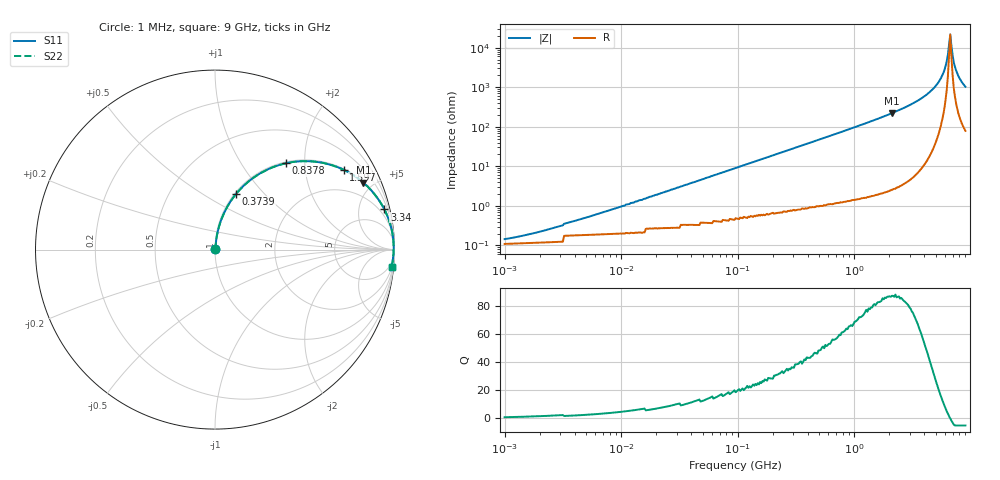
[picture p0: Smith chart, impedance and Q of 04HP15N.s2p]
# MHz S MA R 50
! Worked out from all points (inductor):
!   396 points, 1 MHz to 9 GHz, reference 50 ohm
!   read as one part in series: L = 15 nH near 6.037 MHz
!   highest Q = 87 at 2.107 GHz (marker M1), where L = 16.7 nH
!   self-resonance near 6.518 GHz
!   S11 on the Smith chart (normalised r, x): 1 MHz: 1.00, +0.00; 373.9 MHz: 1.02, +0.71; 837.8 MHz: 1.03, +1.60; 1.597 GHz: 1.04, +3.19; 3.34 GHz: 1.11, +8.41; 9 GHz: 3, -21
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1  0.001508 38.6  0.999 -0.1  0.999 -0.1  0.001508 38.6
1.997  0.00231 54.3  0.999 -0.1  0.999 -0.1  0.00231 54.3
4.578  0.004607 69.0  0.998 -0.2  0.998 -0.2  0.004607 69.0
20.961  0.02 81.3  0.997 -1.1  0.997 -1.1  0.02 81.3
95.968  0.09 81.9  0.991 -5.1  0.991 -5.1  0.09 81.9
373.904  0.331 69.3  0.936 -19.3  0.936 -19.3  0.331 69.3
439.375  0.381 66.3  0.916 -22.4  0.916 -22.4  0.381 66.3
837.792  0.621 50.7  0.774 -38.4  0.774 -38.4  0.621 50.7
1597.486  0.843 31.9  0.528 -57.5  0.528 -57.5  0.843 31.9
2011.613  0.898 25.5  0.43 -63.9  0.43 -63.9  0.898 25.5
2106.521  0.907 24.3  0.411 -65.1  0.411 -65.1  0.907 24.3
3340.263  0.97 13.3  0.231 -75.9  0.231 -75.9  0.97 13.3
4612.443  0.99 6.8  0.119 -81.6  0.119 -81.6  0.99 6.8
5546.474  0.995 3.4  0.059 -83.0  0.059 -83.0  0.995 3.4
5943.595  0.995 2.1  0.037 -81.7  0.037 -81.7  0.995 2.1
6224.015  0.996 1.3  0.022 -77.8  0.022 -77.8  0.996 1.3
6369.149  0.996 0.8  0.015 -72.6  0.015 -72.6  0.996 0.8
6669.648  0.995 -0.0  0.004608 0.9  0.004608 0.9  0.995 -0.0
6984.324  0.995 -0.8  0.015 70.6  0.015 70.6  0.995 -0.8
7313.847  0.994 -1.7  0.03 78.1  0.03 78.1  0.994 -1.7
7837.509  0.993 -2.9  0.052 80.5  0.052 80.5  0.993 -2.9
9000  0.988 -5.5  0.096 80.1  0.096 80.1  0.988 -5.5
